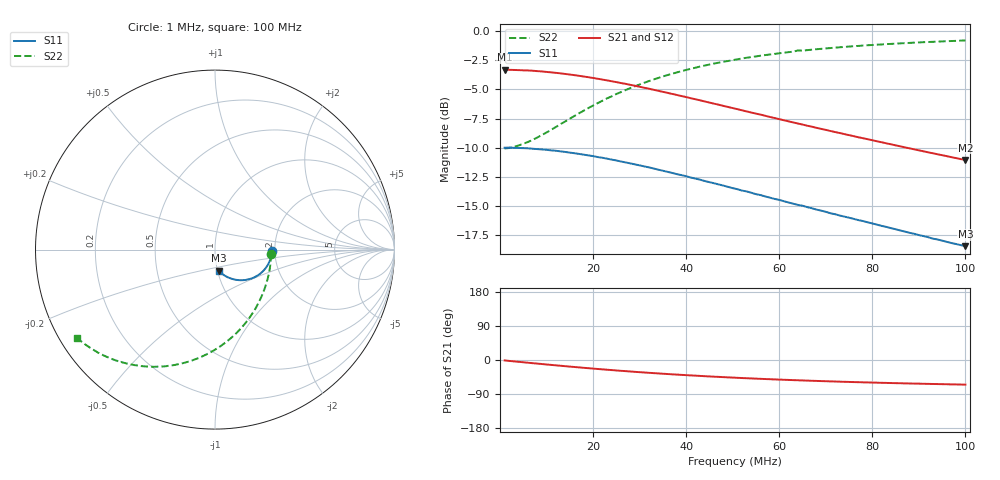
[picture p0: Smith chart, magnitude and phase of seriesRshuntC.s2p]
# Hz S RI R 50.0
! written by SimSmith version 18.3b
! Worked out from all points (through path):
!   100 points, 1 MHz to 100 MHz, reference 50 ohm
!   highest |S21| = -3.31 dB at 1 MHz (marker M1); lowest = -11.0 dB at 100 MHz (marker M2)
!   group delay of S21, straight-line fit = 1.73 ns
!   lowest |S11| = -18.4 dB at 100 MHz (marker M3), VSWR 1.27, Z = 50.6 - j12.1 ohm
!   |S11| at or under -10 dB: 2.973 MHz to end of sweep
!   |S22| runs from -10.1 to -0.8 dB; largest |S21 - S12| = 0.0027
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1000000  0.3165 -0.00634  0.6829 -0.0144  0.6828 -0.0142  0.313 -0.0262
3000000  0.3155 -0.0214  0.6803 -0.0426  0.6804 -0.0427  0.3087 -0.0814
5000000  0.3132 -0.0361  0.6754 -0.0706  0.6754 -0.0706  0.3001 -0.1346
9000000  0.3047 -0.0633  0.6604 -0.1239  0.6599 -0.124  0.2692 -0.237
1.3e7  0.2925 -0.0881  0.6362 -0.1725  0.6361 -0.1725  0.2247 -0.3302
1.8e7  0.2723 -0.115  0.5982 -0.2247  0.5982 -0.2245  0.1517 -0.4303
2.2e7  0.2545 -0.1319  0.5635 -0.2588  0.5635 -0.2585  0.0857 -0.4958
2.5e7  0.24 -0.1427  0.536 -0.28  0.5359 -0.2797  0.0329 -0.5366
2.9e7  0.2203 -0.1537  0.4986 -0.3025  0.499 -0.302  -0.0379 -0.5791
3.4e7  0.1962 -0.1629  0.4524 -0.3216  0.4528 -0.3216  -0.1259 -0.617
3.8e7  0.1775 -0.1673  0.4169 -0.3315  0.4172 -0.3315  -0.1941 -0.6362
4.3e7  0.1559 -0.1704  0.3751 -0.3381  0.3756 -0.3381  -0.2735 -0.6498
5.1e7  0.1246 -0.1694  0.3158 -0.3385  0.3162 -0.3383  -0.3868 -0.6509
5.7e7  0.1041 -0.1657  0.2775 -0.3333  0.278 -0.3334  -0.4607 -0.6411
6.3e7  0.0868 -0.1603  0.244 -0.3248  0.2444 -0.3249  -0.5242 -0.6256
6.4e7  0.0841 -0.1592  0.239 -0.323  0.2403 -0.3253  -0.5371 -0.6281
6.5e7  0.0819 -0.1588  0.2342 -0.3218  0.234 -0.322  -0.5436 -0.6203
6.7e7  0.0765 -0.1567  0.2245 -0.3184  0.2247 -0.3187  -0.5623 -0.6139
7.6e7  0.0565 -0.1464  0.1866 -0.3018  0.1866 -0.302  -0.6347 -0.5828
8.4e7  0.0426 -0.1367  0.1598 -0.2858  0.1599 -0.2862  -0.6861 -0.5531
9.1e7  0.0319 -0.1285  0.1401 -0.2716  0.14 -0.2722  -0.7252 -0.5266
1e8  0.0202 -0.1182  0.1185 -0.2546  0.1182 -0.2549  -0.7666 -0.4936
